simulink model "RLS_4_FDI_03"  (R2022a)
settings: Solver=VariableStepAuto  StartTime=0.0  StopTime=300  RelTol=1e-3
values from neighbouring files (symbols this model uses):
  C = 6.3000e-04    (= 0.00063)    [maglev_init.m]
  g = 9.80    (= 9.8)    [maglev_init.m]
  K = 1.0e+03 * [-2.4567   -0.1235    0.0237]    [maglev_init.m]
  L1 = 0.6000    (= 0.6)    [maglev_init.m]
  m = 0.0300    (= 0.03)    [maglev_init.m]
  mpert = 0    [maglev_init.m]
  R = 45    [maglev_init.m]
  Ts = 0.005    [maglev_init.m]    (also in train_net.m)
  x1_0 = 0.1    [maglev_init.m]
  x1_d = 0.05    [maglev_init.m]
  x2_0 = 0    [maglev_init.m]
  x2_d = 0    [maglev_init.m]
  x3_0 = 0.2    [maglev_init.m]
libraries: ctrlSharedLib x1

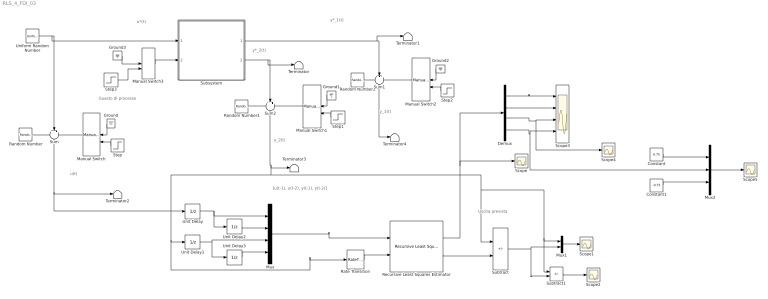
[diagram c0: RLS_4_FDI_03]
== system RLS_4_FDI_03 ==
  note: [u(t-1), u(t-2), y(t-1), y(t-2)]
  note: Uscita prevista
  note: y_2(t)
  note: y*_1(t)
  note: u(t)
  note: y*_2(t)
  note: y_1(t)
  note: u*(t)
  note: Guasto di processo
  Constant : Constant  Value=0.75
  Constant1 : Constant  Value=-0.75
  Demux : Demux
  Ground{,1..3} (4 alike) : Ground
  Manual Switch : ManualSwitch
  Manual Switch1 : ManualSwitch
  Manual Switch2 : ManualSwitch
  Manual Switch3 : ManualSwitch  CurrentSetting=0
  Mux : Mux
  Mux1 : Mux  Inputs=2
  Mux2 : Mux  Inputs=3
  Random Number : RandomNumber  Variance=1e-9  Seed=1  SampleTime=Ts
  Random Number1 : RandomNumber  Variance=1e-6  Seed=3  SampleTime=Ts
  Random Number2 : RandomNumber  Variance=1e-9  Seed=2  SampleTime=Ts
  Rate Transition : RateTransition  OutPortSampleTime=Ts
  Recursive Least Squares Estimator : ctrlSharedLib/Recursive Least Squares Estimator  InitialEstimateSource=None  InitialParameterData=4  P0=1e4  InitialRegressors=0  InitialOutputs=0  History=Infinite  WindowLength=200  EstimationMethod=Forgetting Factor  AdaptationParameter=0.99  HasTimeVaryingAdaptationParameter=off  NormalizationBias=eps  OutputError=on  OutputP=off  AddEnablePort=off  InputProcessing=Sample-based  Ts=Ts
  Scope{,1..2,4..5} (5 alike) : Scope
  Scope3 : Scope  NumInputPorts=4
  Step : Step  Time=150  SampleTime=0
  Step1 : Step  Time=150  SampleTime=0
  Step2 : Step  Time=150  SampleTime=0
  Step3 : Step  Time=150  After=2*R  SampleTime=0
  Subsystem : Subsystem
  Subtract : Sum  Inputs=+-
  Subtract1 : Sum  Inputs=+-
  Sum : Sum  Inputs=+++
  Sum1 : Sum  Inputs=+++
  Sum2 : Sum  Inputs=+++
  Terminator{,1..4} (5 alike) : Terminator
  Uniform Random Number : UniformRandomNumber  Minimum=x1_d*0.9  Maximum=x1_d*1.1  Seed=1  SampleTime=0.5
  Unit Delay{,1..3} (4 alike) : UnitDelay  SampleTime=Ts  HasFrameUpgradeWarning=on
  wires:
  Subsystem/1(Out1) -> Terminator1/1, Sum1/2
  Subsystem/2(Out2) -> Terminator/1, Sum2/2
  Random Number/1 -> Sum/1
  Manual Switch/1 -> Sum/3
  Manual Switch2/1 -> Sum1/3
  Manual Switch1/1 -> Sum2/3
  Random Number1/1 -> Sum2/1
  Ground/1 -> Manual Switch/1
  Step/1 -> Manual Switch/2
  Ground1/1 -> Manual Switch1/1
  Step1/1 -> Manual Switch1/2
  Random Number2/1 -> Sum1/1
  Ground2/1 -> Manual Switch2/1
  Step2/1 -> Manual Switch2/2
  Sum1/1 -> Terminator4/1
  Manual Switch3/1 -> Subsystem/2(fs)
  Ground3/1 -> Manual Switch3/1
  Uniform Random Number/1 -> Subsystem/1(u), Sum/2
  Step3/1 -> Manual Switch3/2
  Sum/1 -> Unit Delay/1, Terminator2/1
  Mux/1 -> Recursive Least Squares Estimator/1
  Rate Transition/1 -> Recursive Least Squares Estimator/2
  Recursive Least Squares Estimator/1 -> Demux/1, Scope/1
  Recursive Least Squares Estimator/2 -> Subtract/2
  Subtract1/1 -> Scope2/1
  Mux1/1 -> Scope1/1
  Subtract/1 -> Subtract1/2, Mux1/2
  Sum2/1 -> Subtract1/1, Mux1/1, Subtract/1, Rate Transition/1, Unit Delay1/1, Terminator3/1
  Unit Delay2/1 -> Mux/2
  Unit Delay/1 -> Unit Delay2/1, Mux/1
  Unit Delay3/1 -> Mux/4
  Unit Delay1/1 -> Unit Delay3/1, Mux/3
  Demux/1 -> Scope3/1
  Demux/2 -> Scope3/2
  Demux/3 -> Scope4/1, Scope3/3
  Demux/4 -> Mux2/2, Scope3/4
  Mux2/1 -> Scope5/1
  Constant/1 -> Mux2/1
  Constant1/1 -> Mux2/3

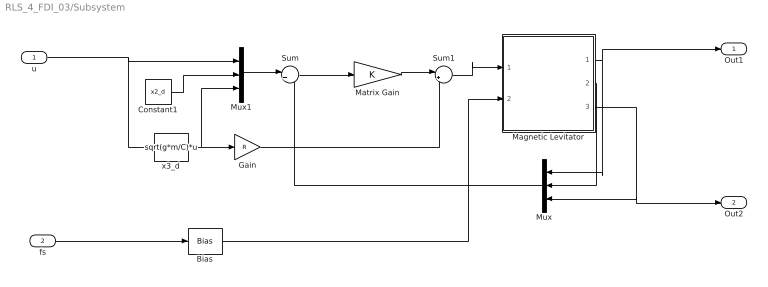
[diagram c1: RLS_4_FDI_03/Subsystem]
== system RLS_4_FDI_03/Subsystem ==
  u : Inport
  fs : Inport  Port=2
  Bias : Bias  Bias=R
  Constant1 : Constant  Value=x2_d
  Gain : Gain  Gain=R
  Magnetic Levitator : Subsystem  mask{m=m+mpert, R=R, L1=L1, C=C, g=g}
      mask prompts: m "ball's mass (m)"; R "Electromagnet's resistance (R)"; L1 "Electromagnet's inductance (L1)"; C "Magnetic force constant (C)"; g "Gravitational acceleration (g)"
  Matrix Gain : Gain  Gain=K  Multiplication=Matrix(K*u)  SaturateOnIntegerOverflow=on
  Mux : Mux  Inputs=3
  Mux1 : Mux  Inputs=3
  Sum : Sum  Inputs=|+-  InputSameDT=on  SaturateOnIntegerOverflow=on
  Sum1 : Sum  Inputs=|++  InputSameDT=on  SaturateOnIntegerOverflow=on
  x3_d : Fcn  Expr=sqrt(g*m/C)*u
  Out1 : Outport
  Out2 : Outport  Port=2
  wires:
  u/1 -> x3_d/1, Mux1/1
  Magnetic Levitator/2(x2) -> Mux/2
  x3_d/1 -> Mux1/3, Gain/1
  Mux1/1 -> Sum/1
  Gain/1 -> Sum1/2
  Mux/1 -> Sum/2
  Constant1/1 -> Mux1/2
  Sum/1 -> Matrix Gain/1
  Sum1/1 -> Magnetic Levitator/1(u)
  Magnetic Levitator/1(x1) -> Out1/1, Mux/1
  Magnetic Levitator/3(x3) -> Out2/1, Mux/3
  Matrix Gain/1 -> Sum1/1
  Bias/1 -> Magnetic Levitator/2(fs)
  fs/1 -> Bias/1

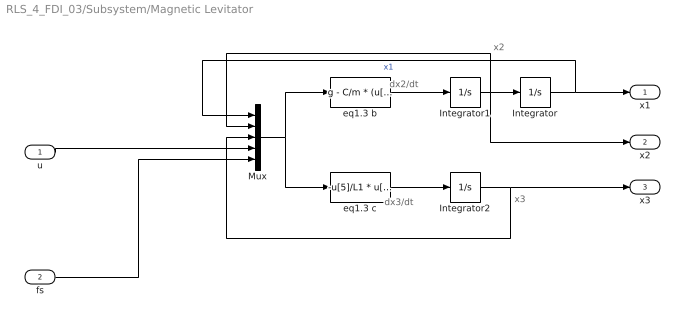
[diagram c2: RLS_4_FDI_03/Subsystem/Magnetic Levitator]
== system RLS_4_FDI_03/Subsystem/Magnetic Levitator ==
  note: x2
  note: x3
  note: dx2/dt
  note: dx3/dt
  u : Inport
  fs : Inport  Port=2
  Integrator : Integrator  InitialCondition=x1_0
  Integrator1 : Integrator  InitialCondition=x2_0
  Integrator2 : Integrator  InitialCondition=x3_0
  Mux : Mux  Inputs=5
  eq1.3 b : Fcn  Expr=g - C/m * (u[3] / u[1])^2
  eq1.3 c : Fcn  Expr=-u[5]/L1 * u[3] + (2*C)/L1 * ( u[2] * u[3] / u[1]^2 ) + 1/L1 * u[4]
  x1 : Outport
  x2 : Outport  Port=2
  x3 : Outport  Port=3
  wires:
  eq1.3 b/1 -> Integrator1/1
  Integrator1/1 -> Integrator/1, Mux/2, x2/1
  eq1.3 c/1 -> Integrator2/1
  Mux/1 -> eq1.3 b/1, eq1.3 c/1
  Integrator/1 -> Mux/1, x1/1  "x1"
  Integrator2/1 -> Mux/3, x3/1
  u/1 -> Mux/4
  fs/1 -> Mux/5
